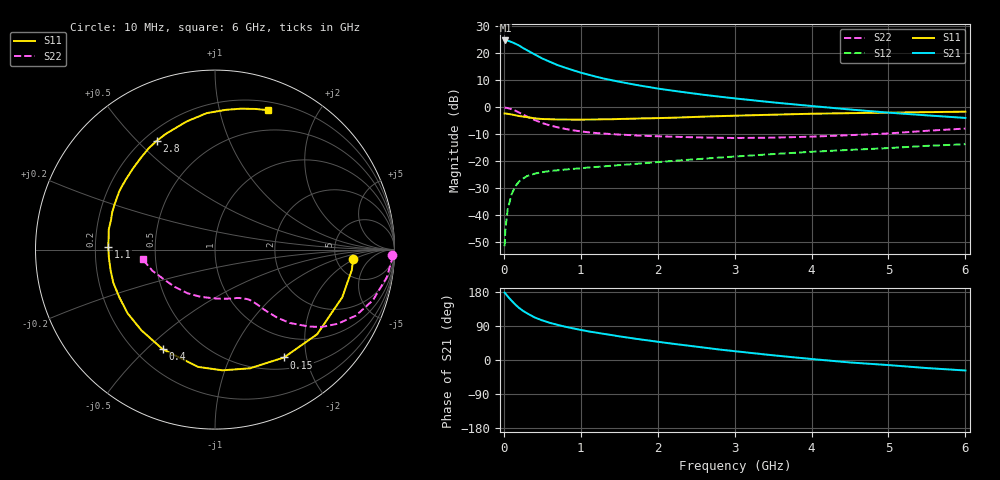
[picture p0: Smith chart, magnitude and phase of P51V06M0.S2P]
! SIEMENS Small Signal Semiconductors
! BFP183
! Si NPN RF Bipolar Junction Transistor in SOT143
! VCE = 1 V  IC = 6 mA
! Common Emitter S-Parameters:  March  1996
# GHz  S  MA  R  50
!  f  S11  S21  S12  S22
! GHz  MAG  ANG  MAG  ANG  MAG  ANG  MAG  ANG
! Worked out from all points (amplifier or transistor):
!   36 points, 10 MHz to 6 GHz, reference 50 ohm
!   highest |S21| = 24.8 dB at 20 MHz (marker M1)
!   |S21| within 3 dB of that: start of sweep to 262.2 MHz
!   unconditionally stable (mu >= 1): 1.353 GHz to end of sweep
!   at 250 MHz: K = 0.25, MSG = 24.1 dB, |S12| = -26.3 dB
!   at 1.4 GHz: K = 1.02, MAG = 15.0 dB, |S12| = -21.6 dB
!   at 6 GHz: K = 1.03, MAG = 3.8 dB, |S12| = -13.7 dB
!   S11 on the Smith chart (normalised r, x): 10 MHz: 7.20, -1.96; 150 MHz: 0.66, -1.62; 400 MHz: 0.31, -0.56; 1.1 GHz: 0.25, +0.01; 2.8 GHz: 0.25, +0.57; 6 GHz: 0.28, +1.41
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0.01  0.7714 -4.1  17.24 177.8  0.0027 87.7  0.989 -1.9
0.02  0.7706 -8.5  17.29 175.6  0.0055 81.9  0.9853 -3.7
0.05  0.7572 -20.5  17.15 167.9  0.013 82.3  0.9701 -9.1
0.1  0.7392 -39.6  16.18 156.6  0.0245 70.0  0.9237 -17.8
0.15  0.7134 -57.4  15.06 146.1  0.0348 62.0  0.8669 -25.1
0.2  0.6895 -73.6  13.89 137.1  0.0426 56.0  0.7993 -31.1
0.25  0.674 -86.4  12.51 129.6  0.0482 50.2  0.735 -35.9
0.3  0.6604 -98.1  11.45 123.5  0.0533 46.3  0.6773 -39.3
0.4  0.6265 -117.8  9.549 112.4  0.0593 40.2  0.583 -44.5
0.5  0.6086 -132.3  8.017 104.5  0.0632 36.3  0.512 -47.6
0.6  0.6026 -144.0  6.952 98.0  0.0665 33.9  0.4626 -49.5
0.7  0.5955 -153.7  6.042 92.6  0.0685 32.5  0.4263 -50.9
0.9  0.5931 -168.6  4.861 83.5  0.0728 31.1  0.3759 -52.9
1.1  0.5951 178.5  4.024 75.5  0.0771 30.8  0.3454 -55.0
1.5  0.6091 160.2  2.981 62.4  0.0854 31.1  0.3138 -59.7
1.8  0.625 148.3  2.487 53.6  0.092 32.1  0.2982 -64.7
2.2  0.643 135.2  2.031 42.8  0.1021 31.7  0.2863 -72.4
2.8  0.6875 118.2  1.579 27.7  0.1178 30.5  0.2738 -86.8
3.5  0.7314 102.4  1.235 12.4  0.1366 28.2  0.2749 -106.5
4.5  0.781 85.6  0.913 -6.5  0.1634 22.5  0.3056 -137.0
5.5  0.8155 73.9  0.711 -21.3  0.194 16.8  0.3686 -161.4
6  0.8314 69.1  0.637 -27.7  0.2077 12.5  0.4053 -172.2
